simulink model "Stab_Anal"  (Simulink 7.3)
settings: Solver=ode45  StartTime=0.0  StopTime=10  RelTol=1e-3
InitFcn:
  | init
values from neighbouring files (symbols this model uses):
  calfa = cos(alfa0*d2r)    [init.m]
  d2r = pi/180    (= 0.0174532925199)    [init.m]    (also in robust.m)
  ge = 32.174    [init.m]
  r2d = 180/pi    (= 57.2957795131)    [init.m]    (also in robust.m)
  salfa = sin(alfa0*d2r)    [init.m]
  Thet0 = 27.69    [init.m]
  V0 = 24675.1    [init.m]
  x0 = [0 0 -2 -2 0 0 18 0 0 0]'*d2r    [init.m]
undefined symbols (not defined in the file or in its folder): As, Bs, Cs, Ds, KmixM0p4, Kpr, Kq

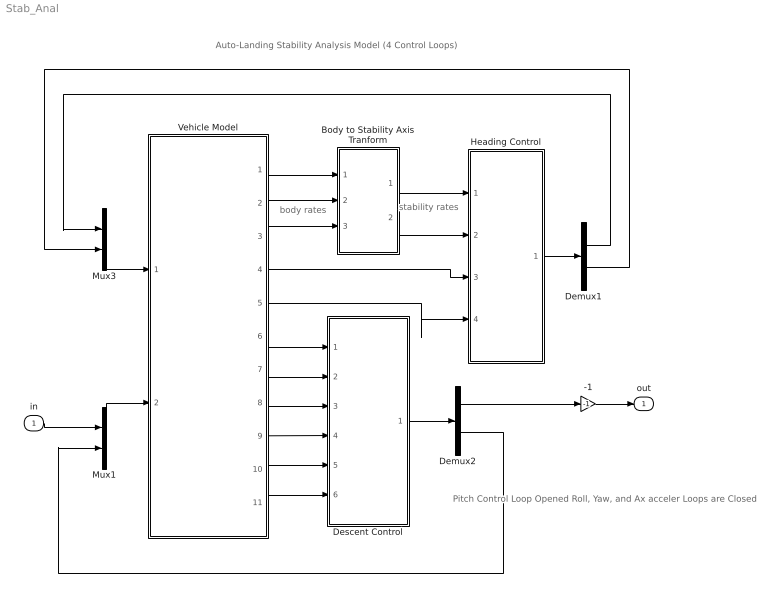
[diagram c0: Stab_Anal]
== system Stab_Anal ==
  note: Auto-Landing Stability Analysis Model (4 Control Loops)
  note: body rates
  note: stability rates
  note: Pitch Control Loop Opened Roll, Yaw, and Ax acceler Loops are Closed
  in : Inport  OutDataType=sfix(16)  OutScaling=2^0
  -1 : Gain  Gain=-1  ParameterDataType=sfix(16)  ParameterScaling=2^0  OutDataType=sfix(16)  OutScaling=2^0
  Body to Stability Axis Tranform : Subsystem
  Demux1 : Demux  Outputs=2
  Demux2 : Demux  Outputs=2
  Descent Control : Subsystem
  Heading Control : Subsystem
  Mux1 : Mux  Inputs=2
  Mux3 : Mux  Inputs=2
  Vehicle Model : Subsystem
  out : Outport  OutDataType=sfix(16)  OutScaling=2^0
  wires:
  Vehicle Model/3(r) -> Body to Stability Axis Tranform/3(r_b)
  Vehicle Model/2(p) -> Body to Stability Axis Tranform/2(p_b)
  Vehicle Model/1(phi) -> Body to Stability Axis Tranform/1(phi)
  Body to Stability Axis Tranform/1(p_s) -> Heading Control/1(ps)
  Body to Stability Axis Tranform/2(r_s) -> Heading Control/2(rs)
  Vehicle Model/5(Vcr) -> Heading Control/4(Vcr)
  Vehicle Model/4(Ny) -> Heading Control/3(Ny)
  Heading Control/1((dP,dR)) -> Demux1/1
  Mux3/1 -> Vehicle Model/1("(dP, dR)")
  Descent Control/1((dQ  dV)) -> Demux2/1
  Mux1/1 -> Vehicle Model/2("(dQ, dV)")
  -1/1 -> out/1
  Demux1/1 -> Mux3/1
  Demux1/2 -> Mux3/2
  Vehicle Model/6(theta) -> Descent Control/1(theta)
  Vehicle Model/7(q) -> Descent Control/2(q)
  Vehicle Model/8(dH) -> Descent Control/3(dH)
  Vehicle Model/9(dV) -> Descent Control/4(Vel)
  Vehicle Model/10(Nz) -> Descent Control/5(Nz)
  Vehicle Model/11(h-dot) -> Descent Control/6(hdot)
  Demux2/1 -> -1/1
  in/1 -> Mux1/1
  Demux2/2 -> Mux1/2

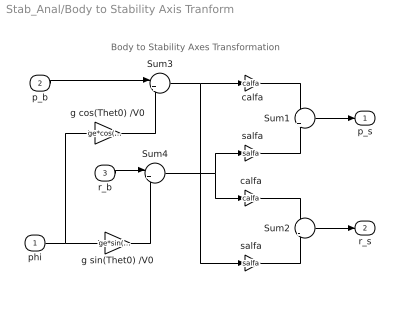
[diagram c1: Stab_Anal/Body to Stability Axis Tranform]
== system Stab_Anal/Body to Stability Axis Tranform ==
  note: Body to Stability Axes Transformation
  phi : Inport  OutDataType=sfix(16)  OutScaling=2^0
  p_b : Inport  Port=2  OutDataType=sfix(16)  OutScaling=2^0
  r_b : Inport  Port=3  OutDataType=sfix(16)  OutScaling=2^0
  Sum1 : Sum  Inputs=+|+  OutDataType=sfix(16)  OutScaling=2^0
  Sum2 : Sum  Inputs=+|-  OutDataType=sfix(16)  OutScaling=2^0
  Sum3 : Sum  Inputs=|++  OutDataType=sfix(16)  OutScaling=2^0
  Sum4 : Sum  Inputs=|+-  OutDataType=sfix(16)  OutScaling=2^0
  calfa : Gain  Gain=calfa  ParameterDataType=sfix(16)  ParameterScaling=2^0  OutDataType=sfix(16)  OutScaling=2^0
  "calfa " : Gain  Gain=calfa  ParameterDataType=sfix(16)  ParameterScaling=2^0  OutDataType=sfix(16)  OutScaling=2^0
  g cos(Thet0) /V0 : Gain  Gain=ge*cos(Thet0*d2r)/V0  ParameterDataType=sfix(16)  ParameterScaling=2^0  OutDataType=sfix(16)  OutScaling=2^0
  g sin(Thet0) /V0 : Gain  Gain=ge*sin(Thet0*d2r)/V0  ParameterDataType=sfix(16)  ParameterScaling=2^0  OutDataType=sfix(16)  OutScaling=2^0
  salfa : Gain  Gain=salfa  ParameterDataType=sfix(16)  ParameterScaling=2^0  OutDataType=sfix(16)  OutScaling=2^0
  "salfa " : Gain  Gain=salfa  ParameterDataType=sfix(16)  ParameterScaling=2^0  OutDataType=sfix(16)  OutScaling=2^0
  p_s : Outport  OutDataType=sfix(16)  OutScaling=2^0
  r_s : Outport  Port=2  OutDataType=sfix(16)  OutScaling=2^0
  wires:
  Sum1/1 -> p_s/1
  Sum2/1 -> r_s/1
  p_b/1 -> Sum3/1
  r_b/1 -> Sum4/1
  g cos(Thet0) /V0/1 -> Sum3/2
  g sin(Thet0) /V0/1 -> Sum4/2
  phi/1 -> g cos(Thet0) /V0/1, g sin(Thet0) /V0/1
  Sum4/1 -> "calfa "/1, salfa/1
  Sum3/1 -> "salfa "/1, calfa/1
  calfa/1 -> Sum1/1
  salfa/1 -> Sum1/2
  "calfa "/1 -> Sum2/1
  "salfa "/1 -> Sum2/2

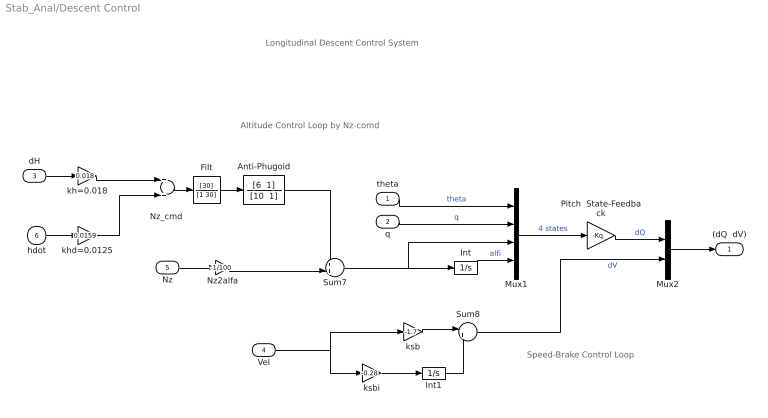
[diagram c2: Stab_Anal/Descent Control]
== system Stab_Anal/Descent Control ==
  note: Speed-Brake Control Loop
  note: Altitude Control Loop by Nz-comd
  note: Longitudinal Descent Control System
  theta : Inport
  q : Inport  Port=2
  dH : Inport  Port=3
  Vel : Inport  Port=4
  Nz : Inport  Port=5
  hdot : Inport  Port=6  OutDataType=sfix(16)  OutScaling=2^0
  Anti-Phugoid : TransferFcn  Numerator="[6  1]"  Denominator="[10  1]"
  Filt : TransferFcn  Numerator=[30]  Denominator=[1 30]
  Int : Integrator
  Int1 : Integrator
  Mux1 : Mux
  Mux2 : Mux  Inputs=2
  Nz2alfa : Gain  Gain=-1/100  ParameterDataType=sfix(16)  ParameterScaling=2^0  OutDataType=sfix(16)  OutScaling=2^0
  "Nz_cmd " : Sum  OutDataType=sfix(16)  OutScaling=2^0
  Pitch  State-Feedback : Gain  Gain=-Kq  Multiplication=Matrix(K*u)  ParameterDataType=sfix(16)  ParameterScaling=2^0  OutDataType=sfix(16)  OutScaling=2^0
  Sum7 : Sum  Inputs=++|  OutDataType=sfix(16)  OutScaling=2^0
  Sum8 : Sum  Inputs=|++  OutDataType=sfix(16)  OutScaling=2^0
  kh=0.018 : Gain  Gain=0.018  ParameterDataType=sfix(16)  ParameterScaling=2^0  OutDataType=sfix(16)  OutScaling=2^0
  khd=0.0125 : Gain  Gain=0.0159  ParameterDataType=sfix(16)  ParameterScaling=2^0  OutDataType=sfix(16)  OutScaling=2^0
  ksb : Gain  Gain=-1.7  ParameterDataType=sfix(16)  ParameterScaling=2^0  OutDataType=sfix(16)  OutScaling=2^0
  ksbi : Gain  Gain=-0.28  ParameterDataType=sfix(16)  ParameterScaling=2^0  OutDataType=sfix(16)  OutScaling=2^0
  (dQ  dV) : Outport
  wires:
  kh=0.018/1 -> "Nz_cmd "/1
  Nz2alfa/1 -> Sum7/2
  Sum8/1 -> Mux2/2  "dV"
  Int1/1 -> Sum8/2
  Nz/1 -> Nz2alfa/1
  Mux2/1 -> (dQ  dV)/1
  ksbi/1 -> Int1/1
  ksb/1 -> Sum8/1
  khd=0.0125/1 -> "Nz_cmd "/2
  hdot/1 -> khd=0.0125/1
  "Nz_cmd "/1 -> Filt/1
  Pitch  State-Feedback/1 -> Mux2/1  "dQ"
  Mux1/1 -> Pitch  State-Feedback/1  "4 states"
  Sum7/1 -> Mux1/3, Int/1
  Int/1 -> Mux1/4  "alfi"
  q/1 -> Mux1/2  "q"
  theta/1 -> Mux1/1  "theta"
  Vel/1 -> ksbi/1, ksb/1
  dH/1 -> kh=0.018/1
  Filt/1 -> Anti-Phugoid/1
  Anti-Phugoid/1 -> Sum7/1

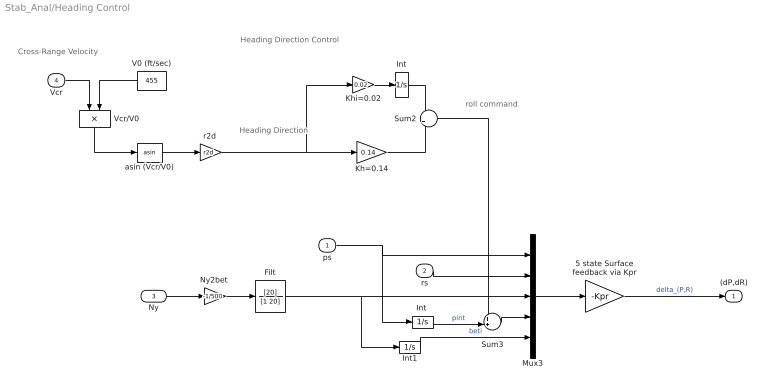
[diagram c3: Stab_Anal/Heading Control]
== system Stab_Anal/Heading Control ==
  note: Heading Direction Control
  note: roll command
  note: Heading Direction
  note: Cross-Range Velocity
  ps : Inport  OutDataType=sfix(16)  OutScaling=2^0
  rs : Inport  Port=2  OutDataType=sfix(16)  OutScaling=2^0
  Ny : Inport  Port=3
  Vcr : Inport  Port=4  OutDataType=sfix(16)  OutScaling=2^0
  5 state Surface feedback via Kpr : Gain  Gain=-Kpr  Multiplication=Matrix(K*u)  ParameterDataType=sfix(16)  ParameterScaling=2^0  OutDataType=sfix(16)  OutScaling=2^0
  Filt : TransferFcn  Numerator=[20]  Denominator=[1 20]
  Int : Integrator
  "Int " : Integrator
  Int1 : Integrator
  Kh=0.14 : Gain  Gain=0.14  ParameterDataType=sfix(16)  ParameterScaling=2^0  OutDataType=sfix(16)  OutScaling=2^0
  Khi=0.02 : Gain  Gain=0.02  ParameterDataType=sfix(16)  ParameterScaling=2^0  OutDataType=sfix(16)  OutScaling=2^0
  Mux3 : Mux  Inputs=5
  "Ny2bet " : Gain  Gain=-1/500  ParameterDataType=sfix(16)  ParameterScaling=2^0  OutDataType=sfix(16)  OutScaling=2^0
  Sum2 : Sum  OutDataType=sfix(16)  OutScaling=2^0
  Sum3 : Sum  Inputs=++|  OutDataType=sfix(16)  OutScaling=2^0
  V0 (ft/sec) : Constant  Value=455  OutDataType=sfix(16)  OutScaling=2^0
  Vcr/V0 : Product  Inputs=*/  OutDataType=sfix(16)  OutScaling=2^0
  asin (Vcr/V0) : Trigonometry  Operator=asin
  "r2d " : Gain  Gain=r2d  ParameterDataType=sfix(16)  ParameterScaling=2^0  OutDataType=sfix(16)  OutScaling=2^0
  (dP,dR) : Outport  OutDataType=sfix(16)  OutScaling=2^0
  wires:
  Vcr/1 -> Vcr/V0/1
  Sum2/1 -> Sum3/1
  Int/1 -> Sum2/1
  Kh=0.14/1 -> Sum2/2
  Khi=0.02/1 -> Int/1
  "r2d "/1 -> Kh=0.14/1, Khi=0.02/1
  Vcr/V0/1 -> asin (Vcr/V0)/1
  asin (Vcr/V0)/1 -> "r2d "/1
  V0 (ft/sec)/1 -> Vcr/V0/2
  Mux3/1 -> 5 state Surface feedback via Kpr/1
  5 state Surface feedback via Kpr/1 -> (dP,dR)/1  "delta_(P,R)"
  rs/1 -> Mux3/2
  ps/1 -> "Int "/1, Mux3/1
  Int1/1 -> Mux3/5  "beti"
  Sum3/1 -> Mux3/4
  "Int "/1 -> Sum3/2  "pint"
  "Ny2bet "/1 -> Filt/1
  Ny/1 -> "Ny2bet "/1
  Filt/1 -> Int1/1, Mux3/3

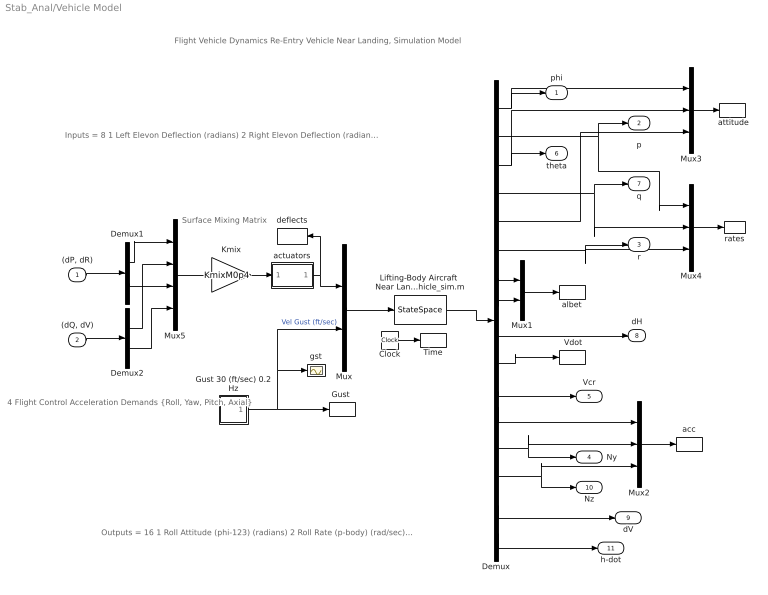
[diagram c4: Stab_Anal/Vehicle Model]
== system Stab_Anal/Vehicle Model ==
  note: Inputs = 8 1 Left Elevon Deflection (radians) 2 Right Elevon Deflection (radians) 3 Vertical Rudder Deflection (radians) 4 Upper Left Body-Flap Deflection (radians) 5 Upper Right Body-Flap Deflection (radians) 6 Lower Left Body-Flap Deflection (radians) 7 Lower Right Body-Flap Deflection (radians) 8 Wind Gust Azim & Elev Angles =(45, 90) (deg)
  note: 4 Flight Control Acceleration Demands {Roll, Yaw, Pitch, Axial}
  note: Outputs = 16 1 Roll Attitude (phi-123) (radians) 2 Roll Rate (p-body) (rad/sec) 3 Pitch Attitude (thet-123) (radians) 4 Pitch Rate (q-body) (rad/sec) 5 Yaw Attitude (psi-123) (radians) 6 Yaw Rate (r-body) (rad/sec) 7 Angle of attack, alfa, (radians) 8 Angle of sideslip, beta, (radian) 9 Change in Altitude, delta-h, (feet) 10 Forward Acceleration (V-dot) (ft/sec) 11 Cross Range Velocity (Vcr) (ft/sec) 12 Accelerom # 1, (along X), (ft/sec^2) Translat. Acceler 13 Accelerom # 2, (along Y), (ft/sec^2) Translat. Acceler 14 Accelerom # 3, (along Z), (ft/sec^2) Translat. Acceler 15 Change in Velocity (delta-V) (ft/sec) 16 Altitude Rate (h-dot) (ft/sec)
  note: Surface Mixing Matrix
  note: Flight Vehicle Dynamics Re-Entry Vehicle Near Landing, Simulation Model
  "(dP, dR)" : Inport  OutDataType=sfix(16)  OutScaling=2^0
  "(dQ, dV)" : Inport  Port=2  OutDataType=sfix(16)  OutScaling=2^0
  " Vdot" : ToWorkspace  VariableName=Vdot  SampleTime=-1  SaveFormat=Array
  " attitude" : ToWorkspace  VariableName=atti  SampleTime=-1  SaveFormat=Array
  Clock : Clock
  Demux : Demux  Outputs=16
  Demux1 : Demux  Outputs=2
  Demux2 : Demux  Outputs=2
  Gust 30 (ft/sec) 0.2 Hz : Subsystem
  "Gust " : ToWorkspace  VariableName=Gust  SampleTime=-1  SaveFormat=Array
  Kmix : Gain  Gain=KmixM0p4  Multiplication=Matrix(K*u)  ParameterDataType=sfix(16)  ParameterScaling=2^0  OutDataType=sfix(16)  OutScaling=2^0
  "Lifting-Body Aircraft  Near Landing,  Simulation Model  from file vehicle_sim.m" : StateSpace  A=As  B=Bs  C=Cs  D=Ds  X0=x0
  Mux : Mux  Inputs=[7,1]
  Mux1 : Mux  Inputs=2
  Mux2 : Mux  Inputs=3
  Mux3 : Mux  Inputs=3
  Mux4 : Mux  Inputs=3
  Mux5 : Mux
  Time : ToWorkspace  VariableName=time  SampleTime=-1  SaveFormat=Array
  acc : ToWorkspace  VariableName=acc  SampleTime=-1  SaveFormat=Array
  actuators : Subsystem
  albet : ToWorkspace  VariableName=albet  SampleTime=-1  SaveFormat=Array
  deflects : ToWorkspace  VariableName=Surf  SampleTime=-1  SaveFormat=Array
  gst : Scope
  rates : ToWorkspace  VariableName=pqr  SampleTime=-1  SaveFormat=Array
  phi : Outport  OutDataType=sfix(16)  OutScaling=2^0
  p : Outport  Port=2  OutDataType=sfix(16)  OutScaling=2^0
  r : Outport  Port=3  OutDataType=sfix(16)  OutScaling=2^0
  Ny : Outport  Port=4  OutDataType=sfix(16)  OutScaling=2^0
  Vcr : Outport  Port=5  OutDataType=sfix(16)  OutScaling=2^0
  theta : Outport  Port=6  OutDataType=sfix(16)  OutScaling=2^0
  q : Outport  Port=7  OutDataType=sfix(16)  OutScaling=2^0
  dH : Outport  Port=8  OutDataType=sfix(16)  OutScaling=2^0
  dV : Outport  Port=9  OutDataType=sfix(16)  OutScaling=2^0
  Nz : Outport  Port=10  OutDataType=sfix(16)  OutScaling=2^0
  h-dot : Outport  Port=11  OutDataType=sfix(16)  OutScaling=2^0
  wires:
  Demux/16 -> h-dot/1
  "(dQ, dV)"/1 -> Demux2/1
  "(dP, dR)"/1 -> Demux1/1
  Demux2/2 -> Mux5/4
  Demux2/1 -> Mux5/2
  Demux1/2 -> Mux5/3
  Demux1/1 -> Mux5/1
  Mux5/1 -> Kmix/1
  Demux/10 -> " Vdot"/1
  Mux4/1 -> rates/1
  Mux3/1 -> " attitude"/1
  Demux/11 -> Vcr/1
  Mux2/1 -> acc/1
  Demux/14 -> Nz/1, Mux2/3
  Demux/13 -> Ny/1, Mux2/2
  Demux/12 -> Mux2/1
  Demux/15 -> dV/1
  Demux/9 -> dH/1
  Mux1/1 -> albet/1
  Demux/7 -> Mux1/1
  Demux/8 -> Mux1/2
  Demux/6 -> Mux4/3, r/1
  Demux/4 -> Mux4/2, q/1
  Demux/2 -> Mux4/1, p/1
  Demux/5 -> Mux3/3
  Demux/3 -> Mux3/2, theta/1
  Demux/1 -> Mux3/1, phi/1
  actuators/1(out) -> deflects/1, Mux/1
  Kmix/1 -> actuators/1(In)
  "Lifting-Body Aircraft  Near Landing,  Simulation Model  from file vehicle_sim.m"/1 -> Demux/1
  Clock/1 -> Time/1
  Gust 30 (ft/sec) 0.2 Hz/1(Gust) -> Mux/2, gst/1, "Gust "/1  "Vel Gust (ft/sec)"
  Mux/1 -> "Lifting-Body Aircraft  Near Landing,  Simulation Model  from file vehicle_sim.m"/1

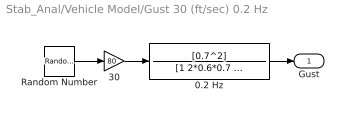
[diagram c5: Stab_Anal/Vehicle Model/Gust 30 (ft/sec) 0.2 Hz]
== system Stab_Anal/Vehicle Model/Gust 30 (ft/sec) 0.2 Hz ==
  0.2 Hz : TransferFcn  Numerator=[0.7^2]  Denominator="[1 2*0.6*0.7  0.7^2]"
  30 : Gain  Gain=80  ParameterDataType=sfix(16)  ParameterScaling=2^0  OutDataType=sfix(16)  OutScaling=2^0
  Random Number : RandomNumber  SampleTime=0
  Gust : Outport  OutDataType=sfix(16)  OutScaling=2^0
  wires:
  0.2 Hz/1 -> Gust/1
  Random Number/1 -> 30/1
  30/1 -> 0.2 Hz/1

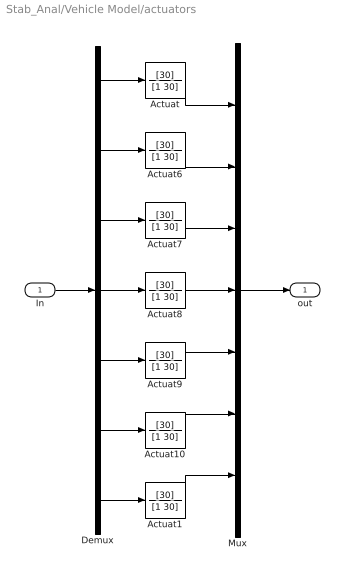
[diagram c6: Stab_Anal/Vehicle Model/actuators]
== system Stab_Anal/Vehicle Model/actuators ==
  In : Inport
  Actuat{,1,6..10} (7 alike) : TransferFcn  Numerator=[30]  Denominator=[1 30]
  Demux : Demux  Outputs=7
  Mux : Mux  Inputs=7
  out : Outport
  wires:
  In/1 -> Demux/1
  Mux/1 -> out/1
  Actuat1/1 -> Mux/7
  Demux/7 -> Actuat1/1
  Demux/1 -> Actuat/1
  Demux/2 -> Actuat6/1
  Demux/3 -> Actuat7/1
  Demux/4 -> Actuat8/1
  Demux/5 -> Actuat9/1
  Demux/6 -> Actuat10/1
  Actuat/1 -> Mux/1
  Actuat6/1 -> Mux/2
  Actuat7/1 -> Mux/3
  Actuat8/1 -> Mux/4
  Actuat9/1 -> Mux/5
  Actuat10/1 -> Mux/6
